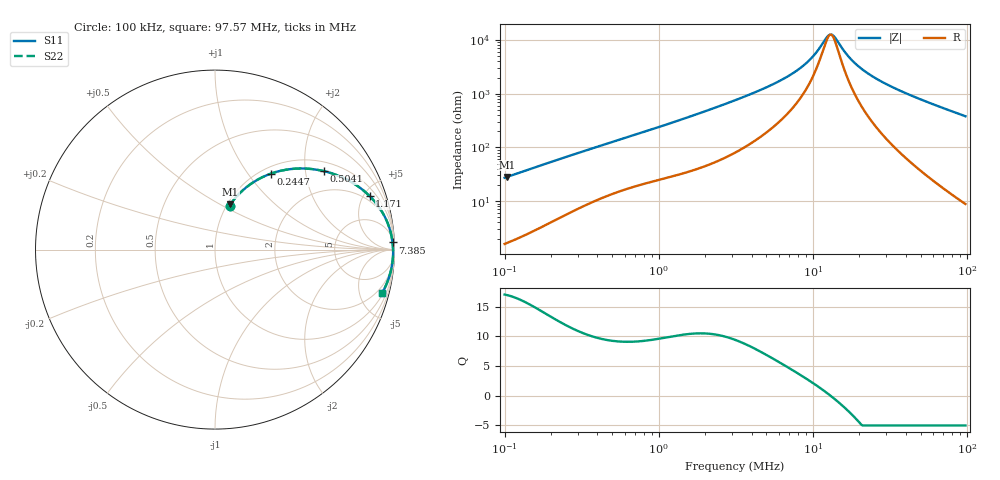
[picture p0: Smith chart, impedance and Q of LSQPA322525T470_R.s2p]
! LSQPA322525T470_R  S-PARAMETER MODEL  ( General Type )
! Model Generated by TAIYO YUDEN Corporation (http://www.ty-top.com)
! Version 2.0
! TAIYO YUDEN Control No. 100810NF25SB-FAC
! Copyright(c) 2007 TAIYO YUDEN CO.,LTD. All Rights Reserved.
! Product Description (link to TY-COMPAS)
! https://ds.yuden.co.jp/TYCOMPAS/or/detail?pn=LSQPA322525T470KR&u=M
! Products Name : Inductors
! Characteristics :
!  Inductance : 47 uH , SRF(min) : 10 MHz , DC Resistance(max) : 0.871 Ohm
!  Rated Current : Saturation :390 mA , Temp Rise : 480 mA (40 degC)
!  Case Size : 3.2 x 2.5 / 0.126 x 0.098 [mm/inch] , Thickness : 2.5 / 0.098 [mm/inch]
!  (Conditions: Temperature = 25 degC , DC Bias Current/Voltage = 0A / 0V)
! External Node Assignments :
!  1  o---GGG---o  2
! GND o---------o GND
! Frequency Range : 0.1MHz  -  97.572838MHz  [ 402 STEP ]
# MHz S RI R 50
! Freq[MHz].  S11 Real  S11 Imag  S21 Real  S21 Imag  S12 Real  S12 Imag  S22 Real  S22 Imag
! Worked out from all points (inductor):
!   401 points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, 100 kHz to 97.57 MHz, reference 50 ohm
!   read as one part in series: L = 43.1 uH near 103.5 kHz
!   highest Q = 16.9 at 103.5 kHz (marker M1), where L = 43.2 uH
!   self-resonance near 12.81 MHz
!   S11 on the Smith chart (normalised r, x): 100 kHz: 1.03, +0.54; 244.7 kHz: 1.11, +1.30; 504.1 kHz: 1.27, +2.53; 1.171 MHz: 1.56, +5.53; 7.385 MHz: 12, +46; 97.57 MHz: 1.18, -7.61
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0.1  0.0814 0.2456  0.9186 -0.2456  0.9186 -0.2456  0.0814 0.2456
0.103502  0.0862 0.2526  0.9138 -0.2526  0.9138 -0.2526  0.0862 0.2526
0.15914  0.1718 0.3449  0.8282 -0.3449  0.8282 -0.3449  0.1718 0.3449
0.244688  0.3114 0.4232  0.6886 -0.4232  0.6886 -0.4232  0.3114 0.4232
0.316747  0.4152 0.4479  0.5848 -0.4479  0.5848 -0.4479  0.4152 0.4479
0.504072  0.6066 0.4373  0.3934 -0.4373  0.3934 -0.4373  0.6066 0.4373
1.003287  0.8276 0.3291  0.1724 -0.3291  0.1724 -0.3291  0.8276 0.3291
1.171346  0.862 0.298  0.138 -0.298  0.138 -0.298  0.862 0.298
1.832278  0.9309 0.2104  0.0691 -0.2104  0.0691 -0.2104  0.9309 0.2104
3.177882  0.9705 0.124  0.0295 -0.124  0.0295 -0.124  0.9705 0.124
5.234367  0.9845 0.0689  0.0155 -0.0689  0.0155 -0.0689  0.9845 0.0689
7.384661  0.989 0.04  0.011 -0.04  0.011 -0.04  0.989 0.04
9.894118  0.9911 0.0188  0.00892 -0.0188  0.00892 -0.0188  0.9911 0.0188
12.37457  0.992 0.00346  0.00798 -0.00346  0.00798 -0.00346  0.992 0.00346
13.25634  0.9922 -0.00124  0.00779 0.00124  0.00779 0.00124  0.9922 -0.00124
13.95865  0.9923 -0.00478  0.00769 0.00478  0.00769 0.00478  0.9923 -0.00478
16.86747  0.9924 -0.0181  0.00756 0.0181  0.00756 0.0181  0.9924 -0.0181
19.35694  0.9922 -0.0282  0.00776 0.0282  0.00776 0.0282  0.9922 -0.0282
23.79669  0.9914 -0.0445  0.0086 0.0445  0.0086 0.0445  0.9914 -0.0445
31.33933  0.9889 -0.0693  0.0111 0.0693  0.0111 0.0693  0.9889 -0.0693
51.61976  0.9772 -0.1284  0.0228 0.1284  0.0228 0.1284  0.9772 -0.1284
97.57284  0.9304 -0.2431  0.0696 0.2431  0.0696 0.2431  0.9304 -0.2431
